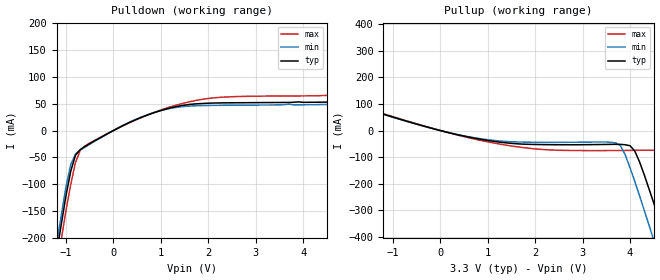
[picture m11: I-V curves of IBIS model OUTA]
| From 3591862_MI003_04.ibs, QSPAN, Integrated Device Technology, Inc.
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|   Model OUTA
[Model]   OUTA
Model_type   Output
Polarity   Non-Inverting
C_comp   5.00pF   5.00pF   5.00pF
[Voltage Range]   3.3000V   3.0000V   4.0000V
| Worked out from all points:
|   slope of the pulldown table from 0 to 0.495 V, typ, clamps not added: 23.4 ohm
|   slope of the pullup table from 0 to 0.495 V, typ, clamps not added: 23.7 ohm
[Pulldown]
| voltage   I(typ)   I(min)   I(max)
-3.3V     -1.425A    -1.409A    -1.452A
-1.5V     -391.2mA   -373.3mA   -420.2mA
-1V       -121mA     -104.5mA   -148.8mA
-900mV    -75.73mA   -63.35mA   -100.2mA
-800mV    -45.9mA    -43.79mA   -59.59mA
-600mV    -29.7mA    -31.03mA   -28.7mA
900mV     34.55mA    34.68mA    35.12mA
2.2V      51.38mA    46.91mA    61.56mA
5.7V      57.63mA    53.63mA    72mA
5.9V      100.9mA    85.37mA    131.2mA
6.1V      184.1mA    167.4mA    215.2mA
6.6V      413.8mA    398.1mA    442.8mA
[Pullup]
| voltage   I(typ)   I(min)   I(max)
-3.3V     355.9mA    223.3mA    694.7mA
-2.9V     195.1mA    161.1mA    510.7mA
-2.7V     160.5mA    144.3mA    419.8mA
-2.1V     111.3mA    111mA      163.5mA
-1.7V     88.9mA     88.7mA     92.55mA
1.1V      -40.04mA   -36.63mA   -45.99mA
3.7V      -51.9mA    -46.55mA   -75.21mA
4.1V      -77.13mA   -191.7mA   -74.46mA
4.5V      -272.7mA   -412mA     -74.2mA
4.7V      -383.1mA   -525mA     -89.04mA
5.3V      -722.7mA   -868.4mA   -378.9mA
6.6V      -1.472A    -1.621A    -1.116A
[Ramp]
| variable   typ   min   max
dV/dt_r   1.2666/0.6855n   1.1190/0.7140n   1.6008/0.6089n
dV/dt_f   1.2624/0.4019n   1.1610/0.3824n   1.5210/0.4427n
R_load = 50.0000
| End [Model] OUTA
